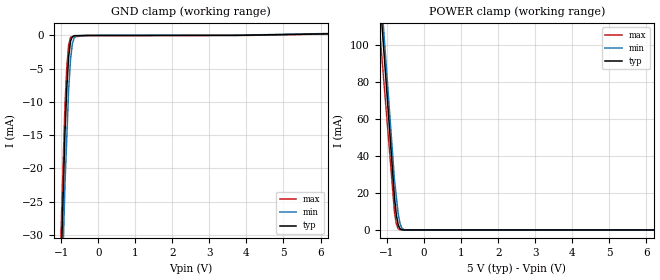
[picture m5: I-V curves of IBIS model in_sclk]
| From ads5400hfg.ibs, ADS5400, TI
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[Model] in_sclk
Model_type Input
Vinl = 800.000mV
Vinh = 2.00000V
C_comp 374.000fF 369.000fF 378.000fF
| variable typ   min   max
[Voltage Range] 5.00000V 4.75000V 5.25000V
[POWER Clamp Reference] 5.00000V 4.75000V 5.25000V
[GND Clamp Reference] 0.00000V 0.00000V 0.00000V
[Temperature Range] 25   85   -40
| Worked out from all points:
|   GND clamp passes 1 mA (typ) near -0.75 V on its own axis
|   POWER clamp passes 1 mA (typ) near -0.66 V on its own axis
[GND Clamp]
-5V       -800.9mA   -838.2mA   -744.6mA
-900mV    -14.81mA   -22.54mA   -10.65mA
-850mV    -7.909mA   -15.35mA   -4.776mA
-800mV    -3.231mA   -8.166mA   -1.439mA
-750mV    -882.9uA   -3.688mA   -277.1uA
-700mV    -181.1uA   -1.247mA   -246.5uA
-650mV    -44.04uA   -366.9uA   -215.9uA
-600mV    -37.99uA   -85.33uA   -185.3uA
-300mV    -4.697uA   -6.314uA   -46.69uA
3.65V     5.206uA    20.68uA    2.304uA
10V       604.7uA    674.4uA    581.6uA
[POWER Clamp]
-5V       1.179A     1.193A     1.046A
-1.05V    86.87mA    96.57mA    71.39mA
-800mV    17.72mA    27.2mA     9.733mA
-750mV    8.256mA    18mA       3.281mA
-700mV    2.793mA    8.799mA    674.6uA
-650mV    632.2uA    3.486mA    126.1uA
-600mV    112.5uA    1.025mA    112uA
-550mV    19.24uA    230.3uA    98.04uA
-400mV    8.747uA    9.405uA    56.02uA
10V       0A         0A         0A
